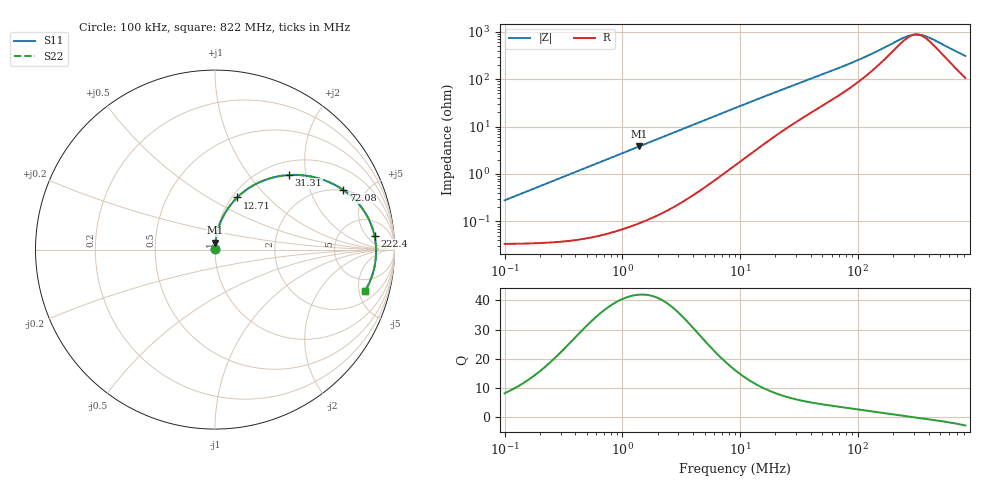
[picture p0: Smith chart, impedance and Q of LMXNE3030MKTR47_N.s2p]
! LMXNE3030MKTR47_N  S-PARAMETER MODEL  ( General Type )
! Model Generated by TAIYO YUDEN Corporation (https://www.yuden.co.jp/en/)
! Version 1.0
! TAIYO YUDEN Control No. 191023NI43SB-FBB
! Copyright(c) 2019 TAIYO YUDEN CO.,LTD. All Rights Reserved.
! Product Description (link to TY-COMPAS)
! https://ds.yuden.co.jp/TYCOMPAS/or/detail?pn=LMXNE3030MKTR47NN&u=M
! Products Name : Inductors
! Characteristics :
!  Inductance : 0.47 uH , SRF(min) : 160 MHz , DC Resistance(max) : 0.0396 Ohm
!  Rated Current : Saturation :2600 mA , Temp Rise : 1900 mA (40 degC)
!  Case Size : 3.0 x 3.0 / 0.118 x 0.118 [mm/inch] , Thickness : 1.2 / 0.047 [mm/inch]
!  (Conditions: Temperature = 25 degC , DC Bias Current/Voltage = 0A / 0V)
! External Node Assignments :
!  1  o---GGG---o  2
! GND o---------o GND
! Frequency Range : 0.1MHz  -  821.96004MHz  [ 402 STEP ]
# MHz S RI R 50
! Freq[MHz].  S11 Real  S11 Imag  S21 Real  S21 Imag  S12 Real  S12 Imag  S22 Real  S22 Imag
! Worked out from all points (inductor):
!   401 points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, 100 kHz to 822 MHz, reference 50 ohm
!   read as one part in series: L = 440 nH near 104.6 kHz
!   highest Q = 41.9 at 1.397 MHz (marker M1), where L = 437 nH
!   self-resonance near 314 MHz
!   S11 on the Smith chart (normalised r, x): 100 kHz: 1.00, +0.01; 12.71 MHz: 1.06, +0.68; 31.31 MHz: 1.27, +1.60; 72.08 MHz: 1.97, +3.45; 222.4 MHz: 11, +8; 822 MHz: 3.13, -5.80
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0.1  0.000342 0.00276  0.9997 -0.00276  0.9997 -0.00276  0.000342 0.00276
0.452624  0.000577 0.0125  0.9994 -0.0125  0.9994 -0.0125  0.000577 0.0125
1.39667  0.00237 0.0382  0.9976 -0.0382  0.9976 -0.0382  0.00237 0.0382
2.048684  0.0045 0.0557  0.9955 -0.0557  0.9955 -0.0557  0.0045 0.0557
4.508421  0.019 0.1201  0.981 -0.1201  0.981 -0.1201  0.019 0.1201
9.272834  0.0722 0.2292  0.9278 -0.2292  0.9278 -0.2292  0.0722 0.2292
12.71254  0.1241 0.2909  0.8759 -0.2909  0.8759 -0.2909  0.1241 0.2909
19.07219  0.2298 0.3666  0.7702 -0.3666  0.7702 -0.3666  0.2298 0.3666
31.31247  0.4108 0.4155  0.5892 -0.4155  0.5892 -0.4155  0.4108 0.4155
41.03579  0.5178 0.4103  0.4822 -0.4103  0.4822 -0.4103  0.5178 0.4103
53.77846  0.6189 0.3828  0.3811 -0.3828  0.3811 -0.3828  0.6189 0.3828
72.08436  0.7135 0.3329  0.2865 -0.3329  0.2865 -0.3329  0.7135 0.3329
113.1315  0.8181 0.2325  0.1819 -0.2325  0.1819 -0.2325  0.8181 0.2325
185.7378  0.878 0.1163  0.122 -0.1163  0.122 -0.1163  0.878 0.1163
222.432  0.8889 0.0757  0.1111 -0.0757  0.1111 -0.0757  0.8889 0.0757
254.6362  0.894 0.0458  0.106 -0.0458  0.106 -0.0458  0.894 0.0458
285.0071  0.8966 0.0212  0.1034 -0.0212  0.1034 -0.0212  0.8966 0.0212
319.0005  0.8976 -0.00346  0.1024 0.00346  0.1024 0.00346  0.8976 -0.00346
349.092  0.8974 -0.0232  0.1026 0.0232  0.1026 0.0232  0.8974 -0.0232
418.0584  0.8941 -0.0634  0.1059 0.0634  0.1059 0.0634  0.8941 -0.0634
671.0681  0.8634 -0.1763  0.1366 0.1763  0.1366 0.1763  0.8634 -0.1763
821.96  0.8369 -0.229  0.1631 0.229  0.1631 0.229  0.8369 -0.229
